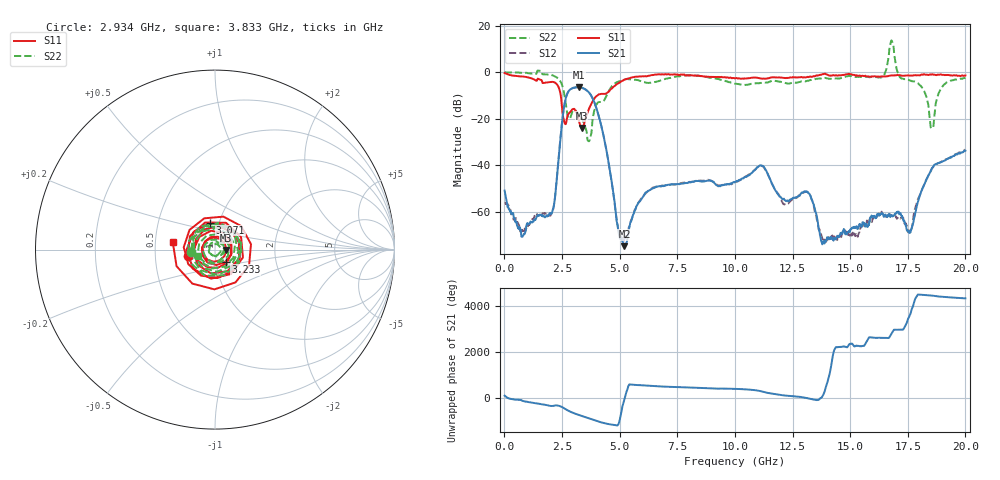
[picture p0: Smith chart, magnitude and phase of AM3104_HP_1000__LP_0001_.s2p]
!Created with skrf (http://scikit-rf.org).
# Hz S RI R 50.0
!freq ReS11 ImS11 ReS21 ImS21 ReS12 ImS12 ReS22 ImS22
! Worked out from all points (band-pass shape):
!   1601 points, 10 MHz to 20 GHz, reference 50 ohm
!   highest |S21| = -6.44 dB at 3.233 GHz (marker M1); lowest = -74.9 dB at 5.207 GHz (marker M2)
!   |S21| within 3 dB of the highest: 2.721 GHz to 3.729 GHz (1.008 GHz wide, 31.3 % of centre)
!   lowest |S11| = -24.0 dB at 3.346 GHz (marker M3), VSWR 1.13, Z = 56.7 - j0.313 ohm
!   |S11| at or under -10 dB: 2.447 GHz to 4.029 GHz (1.582 GHz wide, 48.9 % of centre)
!   |S22| runs from -29.7 to 13.7 dB; largest |S21 - S12| = 0.025
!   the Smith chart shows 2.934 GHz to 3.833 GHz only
!   S11 on the Smith chart (normalised r, x): 2.934 GHz: 0.73, -0.05; 3.071 GHz: 0.91, +0.28; 3.233 GHz: 1.11, -0.15; 3.833 GHz: 0.62, +0.05
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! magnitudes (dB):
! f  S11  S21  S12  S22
! 10 MHz  -0.3  -51.0  -56.3  0.0
! 809.6 MHz  -1.8  -70.4  -68.8  -0.2
! 2.021 GHz  -4.2  -60.8  -61.2  -1.2
! 2.596 GHz  -21.2  -14.5  -14.5  -9.3
! 2.934 GHz  -16.1  -6.9  -7.0  -17.3
! 3.071 GHz  -16.3  -6.5  -6.5  -16.4
! 3.233 GHz  -20.9  -6.4  -6.5  -18.1
! 3.346 GHz  -24.0  -6.6  -6.7  -19.3
! 3.833 GHz  -12.4  -11.3  -11.3  -19.8
! 5.207 GHz  -3.2  -74.9  -71.6  -3.2
! 6.682 GHz  -0.9  -49.1  -49.1  -3.9
! 10.01 GHz  -2.6  -47.3  -47.5  -4.9
! 11.15 GHz  -2.8  -40.2  -40.3  -4.6
! 12.14 GHz  -2.4  -54.8  -56.8  -4.4
! 13.34 GHz  -2.0  -55.1  -54.8  -3.3
! 13.84 GHz  -0.8  -73.1  -71.6  -2.6
! 16.35 GHz  -1.8  -60.8  -60.6  -2.3
! 16.68 GHz  -1.5  -61.3  -62.6  7.2
! 17.6 GHz  -1.4  -68.6  -68.2  -3.5
! 18.54 GHz  -0.9  -41.5  -41.7  -24.2
! 19 GHz  -1.2  -38.5  -38.2  -6.2
! 20 GHz  -1.4  -33.8  -33.4  -2.5
